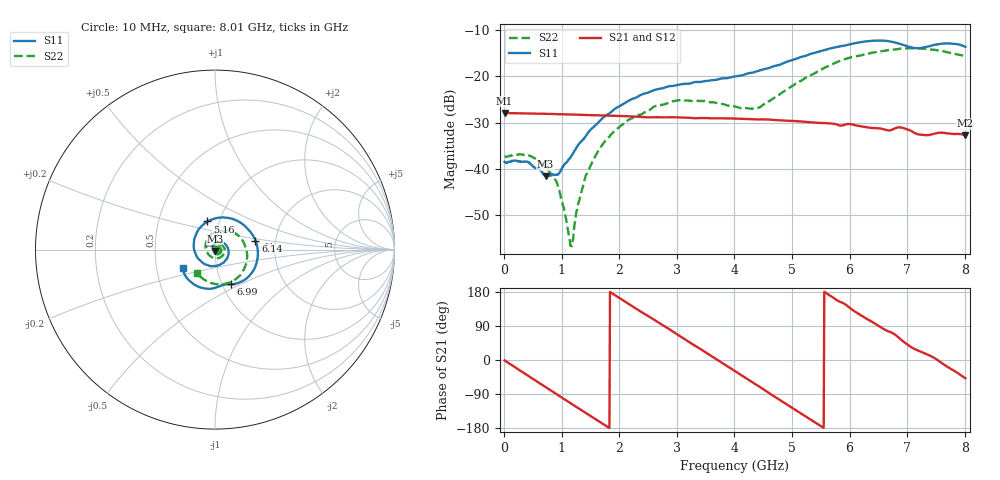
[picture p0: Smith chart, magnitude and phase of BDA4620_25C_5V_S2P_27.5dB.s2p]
!Agilent Technologies,E5071B,MY42404982,A.09.10
!Date: Wed May 06 09:04:27 2026
!Data & Calibration Information:
!Freq	S11:SOLT2(ON)	S21:SOLT2(ON)	S12:SOLT2(ON)	S22:SOLT2(ON)
# Hz S RI R 50
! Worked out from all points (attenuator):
!   801 points, 10 MHz to 8.01 GHz, reference 50 ohm
!   highest |S21| = -27.89 dB at 10 MHz (marker M1); lowest = -32.7 dB at 8.01 GHz (marker M2)
!   lowest |S11| = -41.6 dB at 720 MHz (marker M3), VSWR 1.02, Z = 50 - j0.835 ohm
!   |S11| at or under -10 dB: start of sweep to end of sweep
!   |S22| runs from -56.6 to -13.9 dB; largest |S21 - S12| = 0.0002
!   S11 on the Smith chart (normalised r, x): 10 MHz: 1.02, -0.00; 5.16 GHz: 0.88, +0.28; 6.14 GHz: 1.57, +0.17; 6.99 GHz: 1.10, -0.44; 8.01 GHz: 0.68, -0.15
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1e7  0.0119 -0.000739  0.0403 -0.000807  0.0404 -0.000838  0.0135 -0.000458
4e8  0.00946 -0.00746  0.0306 -0.0255  0.0306 -0.0256  0.0134 -0.00425
7.2e8  3.98e-05 -0.00835  0.0126 -0.0374  0.0126 -0.0374  0.00837 -0.00677
9.4e8  -0.00755 -0.00442  -0.00202 -0.0391  -0.00209 -0.0391  0.0033 -0.0054
1.16e9  -0.0128 0.00459  -0.0161 -0.0353  -0.0161 -0.0353  -0.00128 -0.00077
1.19e9  -0.0133 0.00612  -0.0178 -0.0344  -0.0179 -0.0345  -0.00166 7.68e-05
1.27e9  -0.014 0.0105  -0.0223 -0.0315  -0.0223 -0.0316  -0.00282 0.00235
1.35e9  -0.0138 0.0148  -0.0263 -0.0281  -0.0263 -0.0281  -0.00321 0.00489
1.53e9  -0.0101 0.0256  -0.0332 -0.0188  -0.0332 -0.0188  -0.00297 0.0114
1.77e9  0.00182 0.0377  -0.0376 -0.00411  -0.0376 -0.0041  0.00114 0.0204
2.15e9  0.0333 0.0425  -0.032 0.0189  -0.032 0.019  0.0172 0.0289
2.68e9  0.0729 0.00678  -0.00572 0.0358  -0.00567 0.0358  0.0441 0.0192
3.08e9  0.0694 -0.0442  0.0177 0.0314  0.0179 0.0314  0.0548 -0.00743
4.01e9  -0.0637 -0.0767  0.0305 -0.0172  0.0306 -0.0173  -0.0106 -0.0462
4.42e9  -0.1149 -0.0066  0.0122 -0.0321  0.0122 -0.0321  -0.0443 -0.0125
5.16e9  -0.0424 0.1568  -0.0256 -0.0202  -0.0256 -0.0203  -0.00934 0.0892
5.35e9  0.0117 0.1763  -0.03 -0.0109  -0.0301 -0.0109  0.0232 0.1018
6.14e9  0.2256 0.05  -0.0161 0.0245  -0.0161 0.0246  0.1627 0.0334
6.68e9  0.1836 -0.1539  0.00666 0.0252  0.00668 0.0253  0.1695 -0.0898
6.99e9  0.0872 -0.1935  0.0199 0.0181  0.02 0.0181  0.1263 -0.1559
7.6e9  -0.0686 -0.2144  0.0245 -0.00349  0.0245 -0.00344  -0.0221 -0.1871
8.01e9  -0.1803 -0.1053  0.0154 -0.0173  0.0154 -0.0172  -0.1025 -0.1281
